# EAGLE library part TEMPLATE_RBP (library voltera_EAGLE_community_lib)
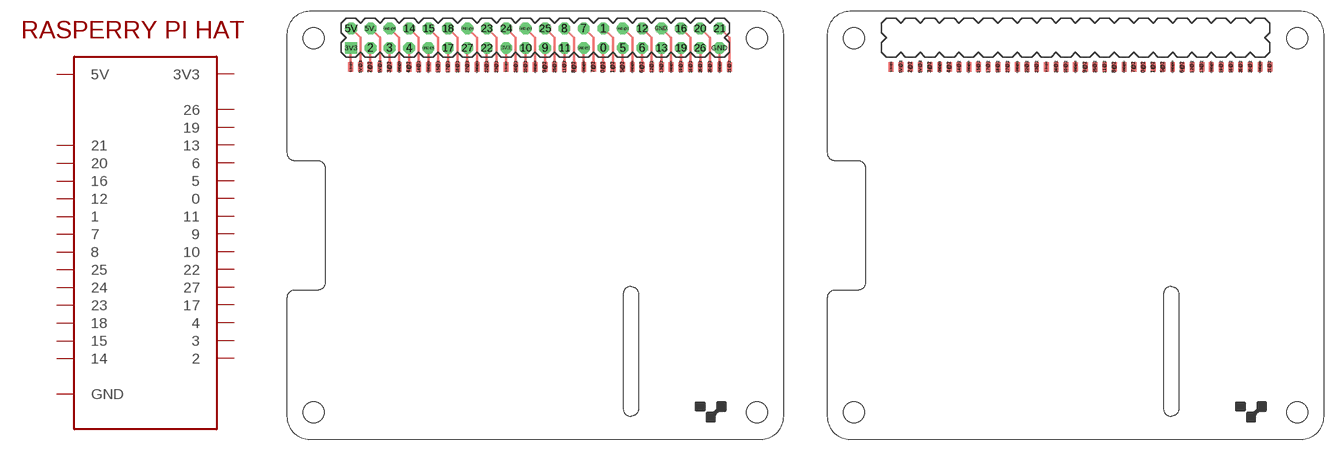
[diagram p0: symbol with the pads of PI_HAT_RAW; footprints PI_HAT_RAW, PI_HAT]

Designator prefix -

## TEMPLATE_RBP_RAW  [PI_HAT_RAW]
0  0
0@1  0
0@2  0
1  1
1@1  1
1@2  1
2  2
2@1  2
2@2  2
3  3
3.3V@1  3V3
3.3V@2  3V3
3.3V@3  3V3
3.3V@4  3V3
3@1  3
3@2  3
3V3  3V3
3V3.  3V3
4  4
4@1  4
4@2  4
5  5
5@1  5
5@2  5
5V  5V
5V.  5V
5V@1  5V
5V@2  5V
5V@3  5V
5V@4  5V
6  6
6@1  6
6@2  6
7  7
7@1  7
7@2  7
8  8
8@1  8
8@2  8
9  9
9@1  9
9@2  9
10  10
10@1  10
10@2  10
11  11
11@1  11
11@2  11
12  12
12@1  12
12@2  12
13  13
13@1  13
13@2  13
14  14
14@1  14
14@2  14
15  15
15@1  15
15@2  15
16  16
16@1  16
16@2  16
17  17
17@1  17
17@2  17
18  18
18@1  18
18@2  18
19  19
19@1  19
19@2  19
20  20
20@1  20
20@2  20
21  21
21@1  21
21@2  21
22  22
22@1  22
22@2  22
23  23
23@1  23
23@2  23
24  24
24@1  24
24@2  24
25  25
25@1  25
25@2  25
26  26
26@1  26
26@2  26
27  27
27@1  27
27@2  27
GND  GND
GND.  GND
GND.@1  GND
GND.@2  GND
GND.@3  GND
GND.@4  GND
GND.@5  GND
GND.@6  GND
GND@1  GND
GND@2  GND
GND@3  GND
GND@4  GND
GND@5  GND
GND@6  GND
GND@7  GND
GND@8  GND
GND@9  GND
GND@10  GND
GND@11  GND
GND@12  GND
GND@13  GND
GND@14  GND
GND@15  GND
GND@16  GND

## TEMPLATE_RBP_SHIELD  [PI_HAT]
0@1  0
0@2  0
1@1  1
1@2  1
2@1  2
2@2  2
3.3V@1  3V3
3.3V@2  3V3
3.3V@3  3V3
3.3V@4  3V3
3@1  3
3@2  3
4@1  4
4@2  4
5@1  5
5@2  5
5V@1  5V
5V@2  5V
5V@3  5V
5V@4  5V
6@1  6
6@2  6
7@1  7
7@2  7
8@1  8
8@2  8
9@1  9
9@2  9
10@1  10
10@2  10
11@1  11
11@2  11
12@1  12
12@2  12
13@1  13
13@2  13
14@1  14
14@2  14
15@1  15
15@2  15
16@1  16
16@2  16
17@1  17
17@2  17
18@1  18
18@2  18
19@1  19
19@2  19
20@1  20
20@2  20
21@1  21
21@2  21
22@1  22
22@2  22
23@1  23
23@2  23
24@1  24
24@2  24
25@1  25
25@2  25
26@1  26
26@2  26
27@1  27
27@2  27
GND@1  GND
GND@2  GND
GND@3  GND
GND@4  GND
GND@5  GND
GND@6  GND
GND@7  GND
GND@8  GND
GND@9  GND
GND@10  GND
GND@11  GND
GND@12  GND
GND@13  GND
GND@14  GND
GND@15  GND
GND@16  GND

## Footprint PI_HAT_RAW (pad centres in mm)
drill 1.016 pad 1.524 octagon: 0 41.39,51.23; 1 41.39,53.77; 2 10.95,51.23; 3 13.45,51.23; 3V3. 28.69,51.23; 4 15.99,51.23; 5 43.93,51.23; 5V 8.41,53.77; 5V. 10.95,53.77; 6 46.47,51.23; 7 38.85,53.77; 8 36.31,53.77; 9 33.77,51.23; 10 31.23,51.23; 11 36.31,51.23; 12 46.47,53.77; 13 49.01,51.23; 14 15.99,53.77; 15 18.53,53.77; 16 51.55,53.77; 17 21.07,51.23; 18 21.07,53.77; 19 51.55,51.23; 20 54.048,53.77; 21 56.59,53.77; 22 26.15,51.23; 23 26.15,53.77; 24 28.69,53.77; 25 33.77,53.77; 26 54.048,51.23; 27 23.61,51.23; GND 56.59,51.23; GND. 49.01,53.77; GND.@1 43.93,53.77; GND.@2 38.85,51.23; GND.@3 31.23,53.77; GND.@4 23.61,53.77; GND.@5 18.53,51.23; GND.@6 13.45,53.77
smd 0.635 x 1.27: 0@1 41.378,48.748; 1@1 42.648,48.748; 2@1 10.898,48.748; 3.3V@1 8.358,48.748; 3.3V@2 28.678,48.748; 3@1 13.438,48.748; 4@1 15.978,48.748; 5@1 43.918,48.748; 5V@1 9.628,48.748; 5V@2 12.168,48.748; 6@1 46.458,48.748; 7@1 40.108,48.748; 8@1 37.568,48.748; 9@1 33.758,48.748; 10@1 31.218,48.748; 11@1 36.298,48.748; 12@1 47.728,48.748; 13@1 48.998,48.748; 14@1 17.248,48.748; 15@1 19.788,48.748; 16@1 52.808,48.748; 17@1 21.058,48.748; 18@1 22.328,48.748; 19@1 51.538,48.748; 20@1 55.348,48.748; 21@1 57.888,48.748; 22@1 26.138,48.748; 23@1 27.408,48.748; 24@1 29.948,48.748; 25@1 35.028,48.748; 26@1 54.078,48.748; 27@1 23.598,48.748; GND@1 14.708,48.748; GND@2 18.518,48.748; GND@3 24.868,48.748; GND@4 32.488,48.748; GND@5 38.838,48.748; GND@6 45.188,48.748; GND@7 50.268,48.748; GND@8 56.618,48.748
smd 0.635 x 1.27 bottom: 0@2 41.378,48.748; 1@2 42.648,48.748; 2@2 10.898,48.748; 3.3V@3 8.358,48.748; 3.3V@4 28.678,48.748; 3@2 13.438,48.748; 4@2 15.978,48.748; 5@2 43.918,48.748; 5V@3 9.628,48.748; 5V@4 12.168,48.748; 6@2 46.458,48.748; 7@2 40.108,48.748; 8@2 37.568,48.748; 9@2 33.758,48.748; 10@2 31.218,48.748; 11@2 36.298,48.748; 12@2 47.728,48.748; 13@2 48.998,48.748; 14@2 17.248,48.748; 15@2 19.788,48.748; 16@2 52.808,48.748; 17@2 21.058,48.748; 18@2 22.328,48.748; 19@2 51.538,48.748; 20@2 55.348,48.748; 21@2 57.888,48.748; 22@2 26.138,48.748; 23@2 27.408,48.748; 24@2 29.948,48.748; 25@2 35.028,48.748; 26@2 54.078,48.748; 27@2 23.598,48.748; GND@9 14.708,48.748; GND@10 18.518,48.748; GND@11 24.868,48.748; GND@12 32.488,48.748; GND@13 38.838,48.748; GND@14 45.188,48.748; GND@15 50.268,48.748; GND@16 56.618,48.748
drill 1.016 pad 1.524 square: 3V3 8.41,51.23
hole 2.75 at 3.5,3.5
hole 2.75 at 61.5,3.5
hole 2.75 at 61.5,52.5
hole 2.75 at 3.5,52.5

## Footprint PI_HAT (pad centres in mm)
smd 0.635 x 1.27: 0@1 41.378,48.748; 1@1 42.648,48.748; 2@1 10.898,48.748; 3.3V@1 8.358,48.748; 3.3V@2 28.678,48.748; 3@1 13.438,48.748; 4@1 15.978,48.748; 5@1 43.918,48.748; 5V@1 9.628,48.748; 5V@2 12.168,48.748; 6@1 46.458,48.748; 7@1 40.108,48.748; 8@1 37.568,48.748; 9@1 33.758,48.748; 10@1 31.218,48.748; 11@1 36.298,48.748; 12@1 47.728,48.748; 13@1 48.998,48.748; 14@1 17.248,48.748; 15@1 19.788,48.748; 16@1 52.808,48.748; 17@1 21.058,48.748; 18@1 22.328,48.748; 19@1 51.538,48.748; 20@1 55.348,48.748; 21@1 57.888,48.748; 22@1 26.138,48.748; 23@1 27.408,48.748; 24@1 29.948,48.748; 25@1 35.028,48.748; 26@1 54.078,48.748; 27@1 23.598,48.748; GND@1 14.708,48.748; GND@2 18.518,48.748; GND@3 24.868,48.748; GND@4 32.488,48.748; GND@5 38.838,48.748; GND@6 45.188,48.748; GND@7 50.268,48.748; GND@8 56.618,48.748
smd 0.635 x 1.27 bottom: 0@2 41.378,48.748; 1@2 42.648,48.748; 2@2 10.898,48.748; 3.3V@3 8.358,48.748; 3.3V@4 28.678,48.748; 3@2 13.438,48.748; 4@2 15.978,48.748; 5@2 43.918,48.748; 5V@3 9.628,48.748; 5V@4 12.168,48.748; 6@2 46.458,48.748; 7@2 40.108,48.748; 8@2 37.568,48.748; 9@2 33.758,48.748; 10@2 31.218,48.748; 11@2 36.298,48.748; 12@2 47.728,48.748; 13@2 48.998,48.748; 14@2 17.248,48.748; 15@2 19.788,48.748; 16@2 52.808,48.748; 17@2 21.058,48.748; 18@2 22.328,48.748; 19@2 51.538,48.748; 20@2 55.348,48.748; 21@2 57.888,48.748; 22@2 26.138,48.748; 23@2 27.408,48.748; 24@2 29.948,48.748; 25@2 35.028,48.748; 26@2 54.078,48.748; 27@2 23.598,48.748; GND@9 14.708,48.748; GND@10 18.518,48.748; GND@11 24.868,48.748; GND@12 32.488,48.748; GND@13 38.838,48.748; GND@14 45.188,48.748; GND@15 50.268,48.748; GND@16 56.618,48.748
hole 2.75 at 3.5,3.5
hole 2.75 at 61.5,3.5
hole 2.75 at 61.5,52.5
hole 2.75 at 3.5,52.5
